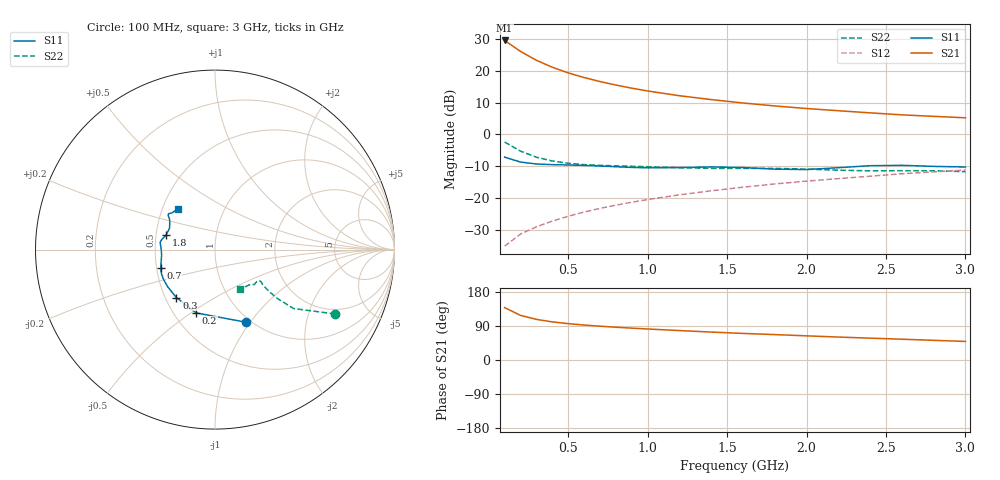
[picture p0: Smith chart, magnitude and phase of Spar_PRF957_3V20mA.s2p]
! Filename:  PRF957G.S2P  Version:  3.0
! NXP part #:  PRF957  Date:  Nov 1998
! Bias condition:  Vce=3V, Ic=20mA
#  MHz  S  MA  R 50
! Freq  S11  S21  S12  S22
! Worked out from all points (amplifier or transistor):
!   20 points, 100 MHz to 3 GHz, reference 50 ohm
!   highest |S21| = 29.6 dB at 100 MHz (marker M1)
!   |S21| within 3 dB of that: start of sweep to 187 MHz
!   unconditionally stable (mu >= 1): 759 MHz to end of sweep
!   at 400 MHz: K = 0.89, MSG = 24.2 dB, |S12| = -27.3 dB
!   at 1.2 GHz: K = 1.05, MAG = 14.3 dB, |S12| = -19.0 dB
!   at 3 GHz: K = 1.03, MAG = 7.1 dB, |S12| = -11.2 dB
!   S11 on the Smith chart (normalised r, x): 100 MHz: 0.95, -0.95; 200 MHz: 0.64, -0.52; 300 MHz: 0.57, -0.35; 700 MHz: 0.53, -0.12; 1.8 GHz: 0.56, +0.10; 3 GHz: 0.60, +0.30
100  0.4396 -66.9  30.13 138.3  0.01748 68.9  0.7594 -28.2
200  0.3681 -106.5  20.25 117.8  0.02714 65.4  0.5468 -36.9
300  0.3431 -128.8  14.69 107.2  0.03524 67.0  0.4388 -38.1
400  0.3351 -142.1  11.42 100.6  0.04338 69.1  0.3824 -37.7
500  0.3311 -150.7  9.313 95.9  0.05167 71.0  0.3521 -37.1
600  0.3262 -156.6  7.864 92.3  0.06012 72.4  0.3354 -36.6
700  0.3191 -161.3  6.801 89.2  0.06867 73.4  0.3263 -36.1
800  0.3108 -165.7  5.991 86.5  0.07719 74.2  0.3208 -35.6
900  0.303 -170.3  5.347 84.0  0.08593 74.8  0.3159 -35.1
1000  0.2987 -174.9  4.834 81.8  0.09465 75.2  0.3109 -34.8
1200  0.3016 177.3  4.068 77.7  0.1123 75.4  0.2999 -35.4
1400  0.3086 172.5  3.539 73.7  0.1298 75.3  0.2929 -37.8
1600  0.3019 169.3  3.127 70.1  0.148 75.1  0.2928 -40.2
1800  0.2848 163.7  2.81 67.0  0.1667 74.5  0.2925 -41.6
2000  0.2803 154.7  2.559 63.7  0.1844 74.0  0.2855 -42.9
2200  0.2998 147.0  2.364 60.5  0.2018 73.4  0.274 -45.7
2400  0.3225 143.9  2.187 57.7  0.2205 72.5  0.2678 -50.0
2600  0.3272 142.5  2.035 54.9  0.2409 71.4  0.2692 -53.8
2800  0.3147 139.3  1.928 51.9  0.2577 70.9  0.2684 -56.0
3000  0.3076 132.1  1.829 49.0  0.2758 70.2  0.2599 -58.2
